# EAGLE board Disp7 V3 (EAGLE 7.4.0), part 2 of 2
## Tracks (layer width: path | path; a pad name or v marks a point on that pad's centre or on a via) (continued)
N$14  (via drill 0.3, 0.5) (continued)
  Top 0.61: R38.2 144.88,94.55 C121.1 145.07,91.5 146.38,91.5 v146.95,90.92 147,90.88 147.01,90.61 147.12,85.5 147.88,84.88 151.75,84.88 153,83.62 v153,81.5 | Q11.4 153.38,21.62 153.38,44.88 157.62,49.12 157.62,80.88 v158.25,81.5
  Route2 0.61: v158.25,81.5 v153,81.5
  AGND$ 0.406: D18.2 v146.95,90.93 v146.95,90.92
N$15
  Top 0.203: 172.78,71.82 C64.2 | 170.4,71.82 IC12.1
  Top 0.305: 170.4,71.82 172.78,71.82
N$16
  Top 0.203: 24.43,91.98 R113.1 | 26.97,91.98 ST6.2 26.97,92.06 | 28.48,96.9 MOD1.P$4
  Top 0.406: 26.97,91.98 24.43,91.98 | 28.48,96.9 28.4,96.42 27.61,92.69 26.97,92.06
N$17
  Top 0.203: R114.1 32.29,91.58 33.08,90.79 42.21,90.79 42.21,91.5 LED2.3
N$18
  Top 0.203: 34.77,91.66 R112.1 | 39.19,93.25 LED2.2
  Top 0.406: 34.77,91.66 36.36,93.25 39.19,93.25
N$19
  Top 0.406: R70.2 R75.2
N$20
  Top 0.203: 40.07,100.08 R110.1 | 42.21,93.33 LED2.4
  Top 0.406: 40.07,100.08 42.21,97.93 42.21,93.33
N$21
  Top 0.406: R71.2 R79.2
N$22  (via drill 0.3)
  Top 0.203: 39.99,101.82 R110.2 | 26.57,111.9 MOD1.P$14
  Top 0.406: v31.42,110.39 39.99,101.82 | v26.89,110.39 26.57,110.71 26.57,111.9
  Route2 0.203: v26.89,110.39 v31.42,110.39
N$23
  Top 0.203: 34.19,93.33 R112.2 | 32.53,96.9 MOD1.P$6
  Top 0.406: 34.19,93.33 33.65,94.5 32.53,96.9
N$24  (via drill 0.3)
  Top 0.203: 18.64,107.3 R109.1 18.72,107.38 18.87,107.38 | 17.05,103.57 ST5.2 | v35.62,110.39 35.62,111.03 36.5,111.9 MOD1.P$9
  Top 0.406: 18.64,107.3 17.05,105.71 17.05,103.57 | 18.87,107.38 v19.92,108.17
  Route2 0.203: v35.62,110.39 33.4,108.17 v19.92,108.17
N$25
  Top 0.203: 26.49,96.03 26.49,96.9 MOD1.P$3 | 24.43,93.96 R111.1
  Top 0.406: 26.49,96.03 24.43,93.96
N$26
  Top 0.203: 32.21,93.33 R114.2 | 30.54,96.9 MOD1.P$5
  Top 0.406: 32.21,93.33 30.92,96.12 30.54,96.9
N$27
  Top 0.254: R36.1 R37.2
  Top 0.406: Q11.1 134.56,18.06 R36.1
N$28
  Top 0.203: 170.4,75.39 170.4,75.55 IC12.4 | 172.78,75.39 C65.2
  Top 0.305: 170.4,75.39 172.78,75.39
N$29
  Top 0.61: JP5.15 142.31,99.69 143.25,98.75 C122.1 R38.1
N$30
  Top 0.203: 170.4,77.06 170.4,76.9 IC12.5 | 172.78,77.06 C65.1
  Top 0.305: 170.4,77.06 172.78,77.06
N$31
  Top 0.203: C58.1 168.89,69.52 168.52,70.02 168.53,72.64 168.53,72.65 168.88,73 170.4,73.01 IC12.2
N$32
  Top 0.203: 172.94,78.64 C57.2 | 170.4,78.17 IC12.6
  Top 0.305: 172.94,78.64 171.51,78.17 170.4,78.17
N$33
  Top 0.61: JP5.1 120.38,97.38 R1.1 C98.1
N$34  (via drill 0.3)
  Top 0.203: v24.91,43.72 21.34,47.29 21.34,47.93 21.97,48.56 21.97,52.45 23,53.48 23,55.39 23.88,56.26 24.25,56.74 26.49,56.74 IC13.47 | v160.48,74.99 163.57,78.09 164.21,78.09 IC12.11 164.29,78.17 | 164.29,79.36 IC12.10
  Top 0.305: 164.29,78.17 164.29,79.36
  Top 0.406: v98.17,45.94 v95.95,43.72
  Route2 0.203: v95.95,43.72 v24.91,43.72 | v98.17,45.94 143.81,45.94 160.48,62.45 v160.48,74.99
N$35  (via drill 0.3)
  Top 0.203: R92.2 C59.2 152.88,91.59 152.97,91.5 153.97,90.76 v153.96,90.64 | 164.21,74.36 IC12.14
  Top 0.305: 164.21,74.36 163.1,74.36 v162.7,74.99
  Route2 0.203: v162.7,74.99 162.7,81.9 v153.96,90.64
N$36
  Top 0.203: 163.89,91.66 Q14.1 | Q13.3 164.29,95.63 | 161.67,96.42 R96.1 161.75,96.42 | 159.21,93.96 159.13,93.96
  Top 0.406: 163.89,91.66 164.37,92.14 Q13.3 | R94.2 159.13,93.96 C53.2 | 159.21,93.96 161.67,96.42 | 164.29,95.63 163.5,96.42 161.75,96.42
N$37  (via drill 0.3)
  Top 0.203: v47.79,62.37 47.77,61.9 47.77,60.25 49.38,58.64 v55.39,58.64 | v109.84,52.61 v104.12,58.32 | v141.35,71.82 152.46,71.82 v152.46,71.98 | 26.57,56.26 IC13.48 34,56.25 34.62,55.62 38.25,55.62 38.8,56.17 v38.8,61.26 | 164.21,76.82 IC12.12
  Top 0.305: v162.07,75.63 163.26,76.82 164.21,76.82
  Route2 0.203: v38.8,61.26 38.85,61.26 39.09,61.02 41.97,61.02 43.32,62.37 v47.79,62.37 | v55.39,58.64 56.34,59.59 102.85,59.59 v104.12,58.32 | v109.84,52.61 122.14,52.61 v141.35,71.82 | v152.46,71.98 152.46,74.36 153.73,75.63 v162.07,75.63
N$38
  Top 0.406: R72.2 R80.2
N$39
  Top 0.203: 163.89,86.74 163.89,86.58 Q16.1 163.89,86.82 | 162.94,89.44 Q14.3
  Top 0.406: 163.89,86.74 R98.1 | 162.94,89.44 163.89,88.49 163.89,86.82
N$40  (via drill 0.3)
  Top 0.203: R99.1 162.94,84.2 Q16.3 162.86,84.2 162.86,83.64 v160,83.64 | v36.65,49.04 36.65,50.8 37.21,51.35 37.21,53.48 IC13.69 | v94.84,53.56 95.71,54.43 103.33,54.43 v103.33,54.51 | v138.57,74.52 142.15,74.58 142.78,75.2 142.78,83.88 143.1,84.2 143.14,84.2 v143.14,84.28
  Route2 0.203: v36.65,49.04 83.49,49.04 88.01,53.56 v94.84,53.56 | v103.33,54.51 104.36,55.55 113.65,55.55 132.62,74.52 v138.57,74.52 | v143.14,84.28 143.65,83.64 v160,83.64
N$41  (via drill 0.3)
  Top 0.203: R93.2 C56.2 156.92,91.59 157.47,91.04 v157.47,89.67 | 169.05,78.33 169.05,79.83 169.85,80.63 170.32,80.63 IC12.8 | 169.05,78.33 169.05,75.63 164.29,75.63 IC12.13 | 169.05,78.33 v168.81,78.33
  Route2 0.203: v168.81,78.33 v157.47,89.67
N$42  (via drill 0.3)
  Top 0.203: v36.58,52.29 36.73,52.45 36.73,53.48 IC13.68 | v115.63,64.75 v114.36,63.48 | 165.8,89.52 Q15.1
  Top 0.305: v42.53,51.81 v40.94,53.4
  Top 0.406: v86.66,57.69 v82.3,53.32 | v107.22,59.2 v105.71,57.69 | v126.43,85.64 133.87,85.64 v134.74,86.79 | 165.8,89.52 v164.84,90.47
  Route2 0.203: v36.58,52.29 37.29,52.29 38.4,53.4 v40.94,53.4 | v42.53,51.81 80.79,51.81 v82.3,53.32 | v105.71,57.69 v86.66,57.69 | v107.22,59.2 111.83,59.2 112,59.38 112,61.25 114.23,63.48 v114.36,63.48 | v115.63,64.75 127,76.25 127.03,79.03 126.91,85.28 126.45,85.53 v126.43,85.64 | v134.74,86.79 136.92,90.09 147.62,90.09 148.65,91.5 163.81,91.5 v164.84,90.47
N$43
  Top 0.203: 169.29,96.42 R97.1 | 166.59,94.76 Q13.1 166.59,94.6 | 166.59,91.82 166.75,91.66 Q15.3
  Top 0.406: 169.29,96.42 166.67,95.07 166.59,94.76 | 166.59,94.6 166.59,91.82
N$44
  Top 0.254: Q4.3 111.22,49.6 R42.2 R29.1
N$45
  Top 0.203: 130.56,40.94 R47.2 | 132.46,40.94 R55.1 132.54,40.94 | 140,42.78 139.93,42.7 Q9.1
  Top 0.406: 132.46,40.94 130.56,40.94 | 140,42.78 134.13,42.78 133.97,42.62 132.54,40.94
N$46  (via drill 0.3)
  Top 0.203: 128.33,91.51 v128.68,91.13
  Top 0.61: R3.2 C103.1 127.64,91.75 v128.68,91.13 128.81,91.12 128.81,88.1 129.76,87.15 v131.51,87.15 | Q9.4 156.43,49.41 v156.43,85.47
  Route2 0.61: v156.43,85.47 156.35,85.39 132.77,85.39 v131.51,87.15
  AGND$ 0.61: v128.68,91.13 127.93,91 D12.2
N$47
  Top 0.203: 181.12,102.3 C119.1 | 181.12,99.76 C117.1 181.04,99.68 | 177.78,100.87 L1.1 | 179.69,95.31 D1.2
  Top 1.016: 181.12,99.76 181.12,100.87 | 181.12,100.87 181.12,102.3 | 177.78,100.87 181.12,100.87 | 179.69,95.31 181.04,96.66 181.04,99.68
N$48
  Top 0.203: R103.1 48.64,64.67 49.91,63.4 52.37,63.4 52.37,61.82 LED1.4
N$49
  Top 0.203: C30.1 76.04,86.67 75.88,86.5 75.88,85.56 IC5.3
  Top 0.406: R82.2 R75.1 C30.1
N$50
  Top 0.61: JP5.3 124.12,97.25 R2.1 C97.1
N$51
  Top 0.203: 127.54,96.38 R3.1
  Top 0.61: JP5.5 R3.1 C96.1
N$52
  Top 0.61: JP5.7 130.12,96.5 | 130.12,96.5 R14.1 | C95.1 130.12,96.5
N$53
  Top 0.203: 74.38,96.62 C18.1
  Top 0.406: JP6.1 75.44,99.44 74.38,98.38 74.38,96.62 | C18.1 R70.1
N$54
  Top 0.406: R73.2 R81.2
N$55  (via drill 0.3)
  Top 0.203: 54.99,79.99 R74.2 | 57.53,79.99 R84.2 57.61,79.99 v60.23,82.61 | 67.88,93.34 R64.2 | 67.93,90.3 C109.1 67.93,90.35
  Top 0.406: 57.53,79.99 54.99,79.99 | 67.93,90.3 67.88,93.34 | 67.93,90.35 67.93,90.3 | 67.93,90.3 v67.93,88.66
  Route2 0.203: v60.23,82.61 61.58,82.61 v67.93,88.66
N$56
  Top 0.61: JP5.9 C94.1 R15.1
N$57
  Top 0.61: JP5.11 135.75,96.88 arc59 C93.1 arc36 R16.1
N$58
  Top 0.203: 41,24.25 40.49,24.25 D3.C
  Top 0.254: JP7.3 49.1,24.89 48.62,25.38 42.12,25.38 41,24.25
N$59
  Top 0.203: 41,22.12 40.5,22.12 D4.C
  Top 0.254: JP7.5 46.56,24.18 46.12,24.62 43.5,24.62 41,22.12
N$60
  Top 0.203: D5.C 41.22,20.13
  Top 0.254: 41.22,20.13 JP7.7
N$61
  Top 0.406: R65.2 R76.2
N$62
  Top 0.406: R66.2 R77.2
N$63
  Top 0.61: JP5.13 139.5,97.38 arc-64 C27.1 R17.1
N$64
  Top 0.203: R83.1 55.37,74.52 56.95,76.1 57.53,76.1 R87.2 57.61,76.18 | 58.8,76.18 C39.1 58.88,76.1
  Top 0.406: 57.61,76.18 58.8,76.18 | R87.2 R84.1 | IC8.3 58.88,75.94 58.88,76.1
N$65
  AGND$ 0.406: R26.1 136.62,90.31 D9.2
N$66
  Top 0.254: U1.8 101.89,74.75 R44.2 R51.2 C47.2
N$67
  Top 0.406: R63.1 60.44,102.81 59.95,103.3 58.95,103.3 C123.1 56.21,106.04 X1.2
N$72  (via drill 0.3)
  Top 0.203: v86.88,87.99 86.7,87.8 86.7,81.03 87.33,80.39 IC7.5 | v90.56,88.04 90.56,89.51 R76.1
  Top 0.406: R76.1 C33.1
  Route2 0.203: v86.88,87.99 v90.56,88.04
N$73
  Top 0.406: JP6.11 89.86,98.64 90.38,98.12 90.38,96.67 R65.1 C86.1
N$75
  Top 0.203: IC9.5 93.69,80.39 92.18,81.9 92.18,87.18 94,89 R77.1
  Top 0.406: C34.1 R77.1
N$76
  Top 0.406: JP6.13 92.41,99.34 93.88,97.88 93.88,96.72 R66.1 C87.1
N$77
  Top 0.406: JP4.1 152,98.12 152.05,98.12 R92.1 C113.2
N$78
  Top 0.203: 56.5,93.49 56.5,93.09 C114.1 | 58.8,93.49 R62.2 58.32,93.41 | IC4.4 61.66,82.93 60.86,82.93 60.55,83.25 C29.1 58.8,83.33 57.77,84.36 57.77,87.38 58.32,87.93 D14.A 58.4,88.01 | 58.4,90.55 D15.C 58.32,90.63
  Top 0.406: 56.5,93.49 58.8,93.49 | 58.4,90.55 58.4,88.01 | 58.32,90.63 58.32,93.41
N$79
  Top 0.203: 61.74,85.55 IC4.3 61.58,85.47 61.58,85.15 | 61.74,88.01 D14.C 61.82,88.09 | C29.2 | 61.82,90.55 D15.A
  Top 0.406: 61.74,88.01 61.74,85.55 | 61.58,85.15 C29.2 | 61.82,90.55 61.82,88.09 64.97,88.09 R52.1 | R63.2 61.75,93.33 | 61.75,93.33 62.78,93.33 C115.1 | D15.A 61.77,93.31 61.75,93.33
N$80
  Top 0.203: 58.8,95.23 R62.1
  Top 0.406: 58.75,95.5 58.56,95.31 R62.1 58.3,96.4 56.42,98.28 56.42,102.78 55.83,103.38 54.16,103.38 C28.1 51.13,106.41 X1.1
N$81
  Top 0.203: 68.53,95.23 R64.1
  Top 0.406: R64.1 67.88,95.97 66.55,97.3 66.55,102.62 65.88,103.3 | 65.88,103.3 64.6,103.3 C110.1 | X1.4 66.37,103.8 65.88,103.3
N$82  (via drill 0.3)
  Top 0.203: R86.2 101.09,88.84 v101.07,88.82
  Top 0.406: v101.09,93.84 R69.2 | IC8.5 68.96,74.67 v68.96,77.06 | v70.86,78.01 71.26,78.41 v73.76,79.68 | C32.1 R86.2
  Route2 0.203: 101.08,89.7 v101.07,88.82 | v101.09,93.84 101.1,92.7 101.1,89.3 v101.07,88.82 | v68.96,77.06 69.91,78.01 v70.86,78.01 | v73.76,79.68 90.29,79.68 v94.5,83.88 | v101.07,88.82 100.25,88.25 94.75,88.25 v94.56,88.32
  Route3 0.203: v94.56,88.32 v94.5,83.88
N$83
  Top 0.406: JP6.17 99.81,98.06 100.25,97.75 100.5,97.38 101.25,96.62 101,96.67 R69.1 C107.1
N$84
  Top 0.406: JP4.3 155.59,99.44 R93.1 C112.2
N$85
  Top 0.203: IC7.3 88.61,89.5 C38.1
  Top 0.406: C38.1 R81.1
N$86
  Top 0.406: JP6.9 87.33,96.97 R73.1 C85.1
N$87
  Top 0.406: JP4.5 157.86,99.23 157.38,98.75 157.38,96.59 C111.2 R94.1
N$88
  Top 0.203: 82.89,89.76 R80.1 83.38,89.58 83.38,88.38 82.25,87.25 IC6.3 | 82.81,89.6 83.64,89.6
  Top 0.406: R80.1 C37.1 | 83.64,89.6 82.89,89.68 82.89,89.76
N$89
  Top 0.406: JP6.7 84.78,96.95 | 84.78,96.95 C52.1 | R72.1 84.41,96.58 84.78,96.95
N$90
  Top 0.406: R4.2 C9.1 R18.2
N$91  (via drill 0.3)
  Top 0.203: 77.81,89.76 R79.1 77.73,89.68
  Top 0.406: v77.73,87.14 77.73,89.68 | v74.48,83.88 74.64,83.72 IC5.5 | R79.1 C36.1
  Route2 0.203: v74.48,83.88 v77.73,87.14
N$92
  Top 0.203: JP6.3 79.69,99.44 | 78,96.62 C51.1
  Top 0.406: 79.69,99.44 78,97.75 78,96.62 | C51.1 R71.1
N$94
  Top 0.406: R9.2 C14.1 R23.2
N$95
  Top 0.406: R8.2 C13.1 R22.2
N$98
  Top 0.406: R7.2 C12.1 R21.2
N$99
  Top 0.406: R6.2 C11.1 R20.2
N$100
  Top 0.406: R5.2 C10.1 R19.2
N$101  (via drill 0.3)
  Top 0.203: 34.59,96.9 MOD1.P$7
  Top 0.406: 34.59,96.9 34.59,96.11 v35.46,95.39
  Route2 0.203: v35.46,95.39 45.23,95.39 46.02,96.19 JP47.3
N$102  (via drill 0.3)
  Top 0.203: 36.58,96.9 MOD1.P$8
  Top 0.406: v39.19,94.28 36.58,96.9
  Route2 0.203: v39.19,94.28 45.47,94.28 JP47.5
N$105
  Top 0.203: 20.54,85.15 Q1.2 | 23.16,85.15 R32.1
  Top 0.406: R39.1 R32.1 | 23.16,85.15 20.54,85.15
N$106
  Top 0.203: 51.5,23.08 JP7.1
  Top 0.254: D2.C 50.75,26.25 51.5,25.5 51.5,23.08
N$108
  Top 0.203: IC6.5 80.98,80.39 80.35,81.03 80.35,87.72 81.62,89 C35.1
  Top 0.406: R78.1 C35.1
N$109
  Top 0.203: 131.03,28.88 R46.2 | 132.46,28.88 R54.1 132.54,28.95 | 140.08,30.54 Q8.1
  Top 0.406: 132.46,28.88 131.03,28.88 | 132.54,28.95 134.13,30.54 140.08,30.54
N$110  (via drill 0.3)
  Top 0.61: R2.2 C104.1 | v122.42,90.94 123.33,91.78 C104.1 | Q8.4 142,33.56 v127.22,33.56 | v121.84,87.23 122.48,87.86 122.48,90.96 123.17,91.65 C104.1 | v131.03,44.35 130.95,44.43 v130.95,47.61 | v118.49,50.47 118.17,50.78 v118.17,53.8 | v116.98,56.9 115.87,58.01 v115.87,58.96 | v114.36,61.02 113.01,62.37 v113.01,65.63 | v113.17,69.67 v113.17,72.14
  Route2 0.61: v121.84,87.23 121.9,87.23 122.03,86.23 122.02,81.48 v113.17,72.14 | v127.22,33.56 131.03,37.37 v131.03,44.35 | v130.95,47.61 128.09,50.47 v118.49,50.47 | v118.17,53.8 116.98,54.99 v116.98,56.9 | v115.87,58.96 114.36,60.47 v114.36,61.02 | v113.01,65.63 113.17,65.78 v113.17,69.67
  AGND$ 0.61: D11.2 122.42,90.92 v122.42,90.94
N$111
  Top 0.406: JP6.5 82.25,98.12 81.62,97.5 C89.1 | C89.1 | C89.1 79.73,96.58 R67.1
N$112
  Top 0.406: R78.2 R67.2
N$113  (via drill 0.3)
  Top 0.203: 97.5,88.43 98.92,88.44 v99.36,88.92 R85.2 | 97.5,88.43 95.69,88.42 94.94,87.68 94.95,85.55 IC9.3 | C31.1 97.57,88.5 97.5,88.43
  Top 0.406: R68.2 v99.3,93.9
  Route2 0.203: v99.36,88.92 100,89.38 100,93.25 v99.3,93.9
N$114
  Top 0.406: JP6.15 94.94,99.43 97.38,97 97.38,96.78 C106.1 R68.1
N$115
  Top 0.406: JP8.3 82.03,23.28 83.88,25.12 83.88,26.64 R5.1
N$116
  Top 0.406: JP8.5 79.49,23.11 80.38,24 80.38,26.66 R6.1
N$117
  Top 0.203: C83.2 39.02,50.27 40.44,50.27 C84.2
  Top 0.254: C84.2 40.5,50.75 40.5,51.12 39.25,52.38 IC13.73
N$118
  Top 0.203: 130.56,66.66 R45.2 | 132.46,66.66 R53.1 132.54,66.66 | 139.78,68.01 Q7.1
  Top 0.406: 132.46,66.66 130.56,66.66 | 132.54,66.66 133.89,68.01 139.78,68.01
N$119
  Top 0.406: JP8.7 76.95,26.55 R7.1
N$120
  Top 0.406: JP8.9 74.41,23.71 73.38,24.75 73.38,26.58 R8.1
N$121
  Top 0.406: JP8.11 71.81,22.93 69.88,24.88 69.88,26.54 R9.1
N$122  (via drill 0.3)
  Top 0.61: R1.2 C105.1 119.5,91.75 118.89,91.19 v118.89,90.88 118.89,87.56 122.77,84.55 135.16,84.55 137.65,86.42 v141.1,86.42 | Q7.4 150.58,68.56 153.02,68.56 154.05,69.59 154.05,84.12 151.75,86.42 v150.4,86.42
  Route2 0.61: v150.4,86.42 v141.1,86.42
  AGND$ 0.305: D13.2 v118.89,90.88
N$124
  Top 0.406: R74.1 R83.2
N$125
  Top 0.61: IC3.4 90.55,73.39 C5.1
N$126
  Top 0.254: D2.A 37.12,28.16 | C19.1 38.18,28.18 38.38,28.38 38.38,31.62 37.88,32.12
  Top 0.406: 37.12,28.16 C19.1 | 37.88,32.12 37.4,32.12 R10.1
N$127
  Top 0.254: D3.A 35.25,24.38 34.52,25.11 C17.1 35.55,28.18 35.75,28.38 35.75,31.75 35.25,32.25
  Top 0.406: 35.25,32.25 34.73,32.25 R11.1
N$128
  Top 0.254: D4.A 32.88,22.12 32.06,22.94 32.06,25.7 C16.1 33.05,28.3 33.25,28.5 33.25,31.75 32.88,32.12
  Top 0.406: 32.88,32.12 32.31,32.12 R12.1
N$129
  Top 0.254: D5.A 30.75,20.12 29.48,21.4 29.48,23.7 C20.1 30.43,28.3 30.75,28.62 30.75,31.62 30,32.38
  Top 0.406: 30,32.38 R13.1
N$132  (via drill 0.3)
  Top 0.406: 137.84,91.83 C100.1
  Top 0.61: R16.2 C100.1 138.49,91.73 139.17,91.23 138.54,91.75 139.23,91.2 139.23,88.26 v139.67,87.94 | Q5.4 155.08,60.56 155.08,84.76 151.83,88.01 v150.4,88.01
  Route2 0.61: v150.4,88.01 150.33,87.94 v139.67,87.94
  AGND$ 0.406: R26.2 139.15,87.42 v139.67,87.94
N$134
  Top 0.203: 130.56,54.43 R49.2 | 132.46,54.43 R58.1 132.54,54.43 | 139.71,55.55 Q5.1
  Top 0.406: 132.46,54.43 130.56,54.43 | 132.54,54.43 133.65,55.55 139.71,55.55
N$135  (via drill 0.3)
  Top 0.203: 147.39,78.2 147.54,78.09 Q6.4
  Top 0.61: R17.2 C99.1 142.69,91.78 v142.72,91.74 142.75,91.74 142.75,86.88 144.16,85.42 144.16,83.35 147.39,78.2
  AGND$ 0.61: v142.72,91.74 142.34,91.07 D10.2
N$136
  Top 0.203: R50.2 130.08,78.88 131.98,78.88 R59.1 132.06,78.88 | 139.78,80.55 Q6.1
  Top 0.406: 132.06,78.88 133.73,80.55 139.78,80.55
N$144
  Top 0.203: C46.1 104.68,66.02 105.71,67.06 105.71,69.2 U1.4
N$145
  Top 0.203: C46.2 103.01,67.52 103.17,67.68 103.17,69.2 U1.2
N$146
  Top 0.203: 105.71,74.75 U1.5 105.79,74.67 107.58,74.71 107.7,74.71 107.85,64.83 106.98,63.96 IC10.4
  Top 0.254: C50.2 107.58,74.71
N$147  (via drill 0.3)
  Top 0.203: v103.41,60.94 103.09,61.26 103.09,61.82 102.38,62.53 101.74,62.53 IC10.6 | 98.88,63.62 D16.C
  Top 0.305: IC10.6 99.88,62.62 98.88,63.62
  Route2 0.203: v103.41,60.94 107.3,57.05 R90.3
N$148
  Top 0.406: JP6.19 101.94,99.94 104.5,97.5 R24.2 C108.1
N$149
  Top 0.203: 106.98,61.34 IC10.2
  Top 0.406: R88.2 R89.2 106.98,61.34
N$150
  Top 0.203: 109.36,59.59 R89.1 | 109.84,54.51 R90.1
  Top 0.406: 109.36,59.59 109.84,59.12 109.84,54.51
N$151  (via drill 0.3)
  Top 0.203: v98.81,80.32 98.81,76.26 98.85,76.14 98.94,75.55 D16.A | C49.2 104.73,89.6 v104.64,88.82
  Top 0.406: C49.2 R91.1
  Route2 0.203: v98.81,80.32 98.81,80.29 98.77,86.23 v104.64,88.82
N$153
  Top 0.203: IC13.12 34.75,69.04 34.75,69.67 33.75,71.17 33.75,74.04 33.4,74.52 33.4,76.82 34.67,78.09 OSC1.3
N$154  (via drill 0.3)
  Top 0.203: C81.2 22.13,55.31 22.13,56.74 C82.2 22.13,56.82 v22.13,57.85 | v25.3,55.78 26.49,55.78 IC13.49
  Route2 0.203: v25.3,55.78 23.24,57.85 v22.13,57.85
N$156  (via drill 0.3)
  Top 0.203: 26.26,72.37 C74.2 | 27.68,72.37 C73.1 | 29.19,72.37 R101.2 | 27.84,72.37 C73.1 | v29.75,67.97 29.75,68.96 IC13.22 | 27.45,72.29 C73.1
  Top 0.406: 27.68,72.37 26.26,72.37 | 27.84,72.37 29.19,72.37 | 27.45,72.29 v27.45,71.23
  Route2 0.203: v29.75,67.97 29.75,68.8 v27.45,71.23
N$157  (via drill 0.3)
  Top 0.203: 29.51,77.45 R95.2 | 31.18,77.45 C55.2 31.34,77.37 31.81,76.9 31.81,75.92 33.35,73.88 33.35,70.76 33.72,70.15 33.72,69.04 IC13.14 33.8,68.96 33.8,68.25 33.88,68.17 33.88,65.23 v34.99,64.12
  Top 0.406: 31.18,77.45 29.51,77.45
  Route2 0.203: v34.99,64.12 38.48,60.63 43.48,60.63 44.12,61.26 54.2,61.26 56.42,63.48 56.74,63.48 ST3.5
N$158  (via drill 0.3)
  Top 0.203: ST4.2 47.69,68.4 47.69,66.98 46.97,66.26 R100.2 46.89,66.34 46.89,66.42 45.54,66.42 45.39,66.26 v44.43,66.26 | v40.86,63.72 40.86,64.2 41.97,64.2 IC13.94
  Route3 0.203: v40.86,63.72 41.89,63.72 v44.43,66.26
N$159  (via drill 0.3)
  Top 0.203: v42.05,54.51 42.05,55.23 IC13.76
  Route2 0.203: v42.05,54.51 43.4,55.86 56.74,55.86 ST3.2
N$160  (via drill 0.3)
  Top 0.203: v38.8,54.83 38.8,53.56 IC13.72
  Route2 0.203: v38.8,54.83 39.43,55.47 42.45,55.47 43.24,56.26 52.05,56.26 56.74,60.94 ST3.4
N$161  (via drill 0.3)
  Top 0.203: v43.48,61.58 43.48,61.74 42.05,61.74 IC13.89 | v55.23,63.24 55.7,63.72 55.7,64.99 56.74,66.02 ST3.6
  Route2 0.203: v43.48,61.58 43.88,61.58 44.04,61.74 53.72,61.74 v55.23,63.24
PLUSZWOELF  (via drill 0.3, 0.5)
  Top 0.203: 171.67,96.5 C118.1 | 172.31,100.79 L1.2 | C116.1
  Top 0.406: v170.64,96.5 171.67,96.5 | v172.86,96.74 C116.1
  Top 1.016: 172.31,100.79 v171.04,100.79
  Route3 0.61: v144.75,98 145.12,98.5
  AGND$ 0.61: D13.1 119.58,97.48 v119.62,98.23 | D11.1 122.8,97.69 v122.76,97.94 | D12.1 126.06,97.57 v126.01,97.94 | D9.1 137.37,97.32 v137.42,97.94 | D10.1 141.13,97.82 v141.08,98.07 | D18.1 v144.75,98
  pour Route3 (isolate 0.305, no thermals): 173.42,105.66 162.15,105.5 162.15,98.49 119.11,98.61 119.11,95.91 173.42,95.79
PTT  (via drill 0.3)
  Top 0.203: 124.36,67.21 R33.1 | 134.12,91.72 C101.1
  Top 0.406: 124.36,67.21 125.79,68.64 v125.79,69.52
  Top 0.61: v132.92,90.55 133.59,91.72 134.12,91.72 | C101.1 R15.2
  Route2 0.203: v125.79,69.52 125.79,71.82 132.06,78.09 132.12,78.09 132.12,79.12 130.06,80.98 130.01,87.92 v132.92,90.55
RS  (via drill 0.3)
  Top 0.203: v31.65,52.29 31.73,52.37 31.73,53.48 IC13.58
  Route2 0.203: v31.65,52.29 31.16,51.42 25.07,51.42 24.35,50.7 18.08,50.7 13.95,46.58 11.81,46.58 10.78,45.54 DSP1.7
UBAND  (via drill 0.3)
  Top 0.203: v29.59,70.31 29.27,69.99 29.27,69.04 IC13.23 | 78.44,85.55 IC5.1 | 77.25,85.55 IC5.2
  Top 0.406: IC5.2 v77.17,83.88 | 77.25,85.55 78.44,85.55
  Route2 0.203: v29.59,70.31 30.15,70.31 31.5,71.66 34.19,71.66 37.05,74.52 37.05,75.42 37.62,75.87 52.07,75.87 52.72,75.84 53.34,75.84 55.62,78.01 64.36,78.01 68.48,82.14 75.11,82.14 76.86,83.88 v77.17,83.88
UFWDANT  (via drill 0.3)
  Top 0.203: v25.37,65.31 26.49,65.31 IC13.30 | v47.37,86.42 v40.94,86.42 | v69.91,77.06 v65.63,81.34 | v86.22,77.06 88.61,79.44 IC7.6 88.68,80.31 | 89.88,80.31 IC7.7
  Top 0.305: v21.41,69.2 22.13,69.91 v22.13,73.41
  Top 0.406: v35.15,86.42 v32.77,84.04 | 88.68,80.31 89.88,80.31
  Route2 0.203: v25.37,65.31 24.51,65.31 21.41,68.4 v21.41,69.2 | v32.77,84.04 v22.13,73.41 | v40.94,86.42 v35.15,86.42 | v47.37,86.42 47.77,86.42 49.67,84.52 57.37,84.52 60.55,81.34 v65.63,81.34 | v86.22,77.06 v69.91,77.06
UFWDFLT  (via drill 0.3)
  Top 0.203: v33.24,67.85 33.24,68.96 IC13.15 | v53.38,74.36 v52.61,73.09 | v83.54,83.88 83.53,84.99 IC6.2 83.6,85.55 | 84.8,85.55 IC6.1
  Top 0.406: 83.6,85.55 84.8,85.55
  Route2 0.203: v33.24,67.85 34.57,67.85 38.32,71.6 38.32,72.45 39.19,73.33 52.37,73.33 v52.61,73.09 | v53.38,74.36 56.34,74.36 59.2,77.22 64.67,77.22 68.8,81.34 81,81.34 v83.54,83.88
UFWDIN  (via drill 0.3)
  Top 0.203: v27.68,63.32 27.68,62.77 27.21,62.29 26.57,62.29 IC13.36 | v51.74,72.69 51.81,72.77 v51.81,74.44 | v75.91,81.98 IC5.6 75.98,80.31 | 77.17,80.31 IC5.7
  Top 0.406: 75.98,80.31 77.17,80.31
  Route2 0.203: v27.68,63.32 27.68,64.2 27.37,64.52 27.37,65.15 27.82,65.73 28.77,65.73 30.38,67.21 36.18,67.21 41.89,72.93 51.5,72.93 v51.74,72.69 | v51.81,74.44 52.45,75.07 53.24,75.07 55.78,77.61 64.52,77.61 68.64,81.74 75.67,81.74 v75.91,81.98
UMESS  (via drill 0.3)
  Top 0.203: v28.64,66.49 28.64,65.78 26.57,65.78 IC13.29 | v44.67,71.66 44.68,72.17 44.68,74.55 45.42,75.41 53.75,75.41 v53.75,78.17 | 61.26,77.22 IC8.2 | 60.7,77.93 60.7,77.85 60.66,77.81 | 61.26,78.48 IC8.1
  Top 0.406: 61.26,77.22 60.66,77.81 v59.44,79.04 | 60.7,77.93 61.26,78.48
  Route2 0.203: v29.91,65.78 35.3,65.78 41.89,72.37 42.69,72.37 43.4,71.66 v44.67,71.66 | v53.75,78.17 54.55,79.04 55.55,79.04 v59.44,79.04
  Route3 0.203: v28.64,66.49 29.59,65.78 v29.91,65.78
UREVANT  (via drill 0.3)
  Top 0.203: v28,64.83 28,64.75 26.57,64.75 IC13.31 | v93.84,78.64 94.95,79.75 IC9.6 95.03,80.31 | 96.22,80.31 IC9.7
  Top 0.406: 95.03,80.31 96.22,80.31
  Route2 0.203: v28,64.83 29.11,64.83 29.43,65.15 53.72,65.15 55.31,66.74 55.86,66.74 67.77,78.64 v93.84,78.64
UREVFLT  (via drill 0.3)
  Top 0.203: v32.84,70.15 32.77,70.07 32.77,69.04 IC13.16 | v89.89,83.88 89.88,84.99 IC7.2 89.95,85.55 | 91.14,85.55 IC7.1
  Top 0.406: 89.95,85.55 91.14,85.55
  Route2 0.203: v32.84,70.15 33.48,70.15 37.05,73.72 56.26,73.72 59.36,76.82 64.83,76.82 68.96,80.95 86.95,80.95 v89.89,83.88
UREVIN  (via drill 0.3)
  Top 0.203: v33.24,66.58 32.29,67.91 32.29,68.96 IC13.17 | v37.61,64.12 v35.15,66.58 | v74.99,74.52 75,75.75 75.75,76.5 80.25,76.5 81,77.25 81,78 82.25,79.25 IC6.6 82.33,80.31 | 83.53,80.31 IC6.7
  Top 0.406: 82.33,80.31 83.53,80.31
  Route2 0.203: v35.15,66.58 v33.24,66.58 | v37.61,64.12 38.16,64.12 38.4,64.36 54.43,64.36 54.91,63.88 55.55,63.88 56.66,64.99 57.21,64.99 64.2,71.98 72.45,71.98 v74.99,74.52
UTEMP  (via drill 0.3)
  Top 0.203: v24.8,64.61 25.3,64.28 26.49,64.28 IC13.32 | v24.86,68.96 24.86,75.15 25.5,75.79 v31.18,75.79 | 66.42,75.94 IC8.6 | 65.86,76.66 65.86,76.58 65.83,76.54 | 66.42,77.22 IC8.7
  Top 0.406: v38.16,81.98 v36.02,79.83 | 66.42,75.94 65.83,76.54 v63.32,79.04 | 65.86,76.66 66.42,77.22
  Route2 0.203: v24.8,64.61 26.06,64.62 26.06,68.01 v24.86,68.96 | v31.18,75.79 31.97,75.79 v36.02,79.83 | v38.16,81.98 46.81,81.98 48.96,84.12 55.7,84.12 60.78,79.04 v63.32,79.04
UTEMP2  (via drill 0.3)
  Top 0.203: v32.45,72.29 32.45,70.71 31.81,70.07 31.81,69.04 IC13.18 | v96.24,83.88 96.22,84.99 IC9.2 96.3,85.55 | 97.5,85.55 IC9.1
  Top 0.406: 96.3,85.55 97.5,85.55
  Route2 0.203: v32.45,72.29 32.45,74.2 34.51,76.26 44.2,76.26 45.84,78.03 49.88,78 50.38,77.5 51.5,77.5 54.47,77.53 55.47,78.41 64.2,78.41 68.33,82.53 74.95,82.53 76.54,84.12 76.54,84.2 76.86,84.52 95.6,84.52 v96.24,83.88
VCC  (via drill 0.3)
  Top 0.203: R40.2 120.32,61.42 120.32,60.07 120.08,59.83 R35.1 120,59.75 v119.12,58.88 119.12,57.85 119.6,57.37 D6.C | v38.8,84.68 38.16,84.68 C54.1 | 22.68,94.2 22.68,93.96 R111.2 | v21.97,91.98 22.61,91.98 R113.2 | v44.17,50.19 43.54,50.19 C79.1 | v45.76,50.19 45.05,50.19 C72.2 | v29.4,74.83 29.27,74.12 R101.1 | v29.43,79.75 29.43,79.12 R95.1 | v23.24,89.6 R39.2 | v18.32,109.76 18.32,109.36 18.64,109.04 R109.2 | 161.83,71.34 C61.2 | 169.29,94.76 R97.2 | v50.55,65.78 50.55,64.91 50.62,64.83 LED1.1 | v38.32,91.5 39.19,91.5 LED2.1 | v40.23,83.72 40.23,83.09 39.75,82.61 OSC1.1 | v22.13,113.09 22.13,112.3 22.45,111.98 MOD1.P$16 | v32.13,113.25 32.13,112.3 32.45,111.98 MOD1.P$11 | 164.29,71.74 IC12.16 | v25.94,52.13 25.94,52.61 26.02,52.69 C66.2 | 37.77,70.23 37.75,70.23 | v43.08,69 42.54,70.05 C80.1 | v42.75,50.19 42.11,50.19 C70.2 | v31.5,72.61 31.1,72.21 C76.1 | 25.3,66.26 25.3,66.25 | 35.23,70.15 35.25,70.15 | v178.02,51.42 178.02,51.39
  Top 0.254: IC13.50 26.1,54.85 C77.1 C66.2 | C70.2 42.62,50.62 41.88,51.38 40.25,52.6 IC13.75 | IC13.28 25.3,66.25 24.1,66.25 C68.2 C75.1 | C76.1 31.25,71.9 IC13.19 | C67.2 34.83,72.32 | 34.83,72.32 34.83,71.66 35.25,71.24 35.25,70.15 IC13.11 | C78.1 37.75,71.4 37.75,70.23 IC13.6 | 34.83,72.32 34.91,72.4 | IC13.100 42,67.35 C71.2 C80.1 | v17.81,96.12 C88.2
  Top 0.305: v161.83,70.23 161.83,71.34 | v164.29,70.86 164.29,71.74 | C69.2 v36.89,72.61 | C75.1 v23.4,68.01
  Top 0.406: 34.91,72.4 C69.2 | 22.68,94.2 v23.48,95 | v168.66,84.2 R99.2 | v168.66,86.74 R98.2 | 169.29,94.76 168.1,93.57 v168.1,92.14 | v39.75,79.68 OSC1.4 | C78.1 v38.96,72.14 | R34.2 v29.5,38.06 v29.5,38.07 | R31.2 32.05,37.87 v32.12,38.07 | R30.2 34.59,37.91 v34.62,38.07 | R115.2 37.12,37.94 v37.12,38.07
  Top 1.016: C6.1 178.02,51.39 176.52,51.39 IC1.3
  Route3 0.203: v168.1,92.14 168.02,91.98 | 47.69,71.02 ST4.1
  Route3 0.305: 46.42,71.02 47.69,71.02
  other vias: 22.92,113.09 19.11,109.76 32.92,113.25 21.97,94.04 24.03,68.01
  pour Route3 (isolate 0.305, no thermals): 168.02,91.98 171.04,89.76 171.04,58.01 173.89,55.15 177.39,55.15 183.74,48.8 183.74,29.27 171.04,16.57 25.62,16.57 9.27,32.92 9.27,74.99 13.4,79.12 13.56,114.05 69.75,114.05 70,85.15 46.42,85.15 46.42,67.37 101.58,67.37 arc2 101.63,91.98
VCCIO  (via drill 0.3)
  Top 0.203: v48.96,76.58 C60.1 | v64.2,80.39 C40.1 | v63.56,82.14 63.56,82.85 IC4.5 | v87.69,73.72 87.69,73.41 | v50.7,78.8 50.7,79.28 50.62,79.36 C43.1 | v79.4,77.85 C41.1 | v85.75,77.85 C45.1 | v92.1,77.85 C42.1 | v97.32,77.85 C44.1
  Top 0.406: IC9.8 97.5,78.8 97.46,78.46 C44.1 | IC7.8 91.36,80.11 C42.1 | C45.1 84.8,78.06 IC6.8 | C41.1 78.44,78.06 IC5.8 | IC11.1 48.57,79.54 C43.1 | IC8.8 64.58,80.39 v64.2,80.39
  Top 0.61: C8.1 87.58,73.41 87.69,73.41 IC3.5
  other vias: 88.64,74.52
  pour Route3 (isolate 0.305, no thermals): 48.32,68.64 97.06,68.48 97.06,82.3 48.32,82.45
VREF2  (via drill 0.3)
  Top 0.203: 48.4,82.77 48.24,82.93 C63.2 48.24,83.01 | 48.4,81.34 IC11.2 48.32,81.42 | C62.1 48.24,85.47 48.24,84.76 48.32,84.76 | v30.15,71.26 30.23,71.18 30.23,69.04 IC13.21 | v99.25,92.25 99.25,91.55 R85.1
  Top 0.406: 48.4,81.34 48.4,82.77 | 48.24,83.01 48.24,84.76 | 48.32,81.42 v47.21,81.42 | 48.32,84.76 v49.35,85.79 | R85.1 R86.1
  Route2 0.203: v30.15,71.26 30.15,72.45 34.35,76.66 42.85,76.66 47.21,81.03 v47.21,81.42 | v49.35,85.79 63.3,85.79 63.5,85.88 70.72,93.09 98.41,93.09 v99.25,92.25
WIFI_RXD  (via drill 0.3)
  Top 0.203: v28.64,71.36 28.2,71.17 28.24,69.44 IC13.25
  Top 0.406: v38.24,83.33 v35.38,80.47
  Route2 0.203: v28.64,71.36 28.64,75.15 33.88,80.39 35.3,80.39 v35.38,80.47 | v38.24,83.33 38.8,83.33 47.45,91.98 47.45,95.07 48.56,96.19 JP47.4
WIFI_TXD  (via drill 0.3)
  Top 0.203: v26.49,71.26 26.49,67.29 IC13.26
  Route2 0.203: v26.49,71.26 26.49,73.01 24.99,74.52 24.99,75.15 28.95,79.12 32.05,79.12 33.96,81.03 v34.67,81.03 | v36.34,82.69 40.15,82.69 48.56,91.11 48.56,93.65 JP47.6
  Route3 0.203: v36.34,82.69 v34.67,81.03

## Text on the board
tNames: SH- | SH+ | GND | PS+ | GND | UBAND | IN-FWD | IN-REV | FLT_FWD | FLT_REV | ANT_FWD | ANT_REV | NTC-2 | NTC-1 | ALC | PSoff | ANT-1 | ANT-2 | PTTout | PTTin | FAN | PSon | PS pre. | TxD | RxD | CIV | +12 | RES | 3v3 | GND | PGM | * | BOOT | +12 | PGM | 5V | 3v3 | AGC | GND | Controller / DSP7 V3 / DJ0ABR / / AB5HM | TRX-4 | TRX-3 | TRX-2 | TRX-1 | 6m | 12+10m | 17+15m | 30+20m | 40+60m | 80m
